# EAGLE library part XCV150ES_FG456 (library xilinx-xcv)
xcv150es_fg456 edit this description Auto generated by make-symbol-device-package-bsdl.ulp Rev. 26 Source: xcv150es_fg456.bsd
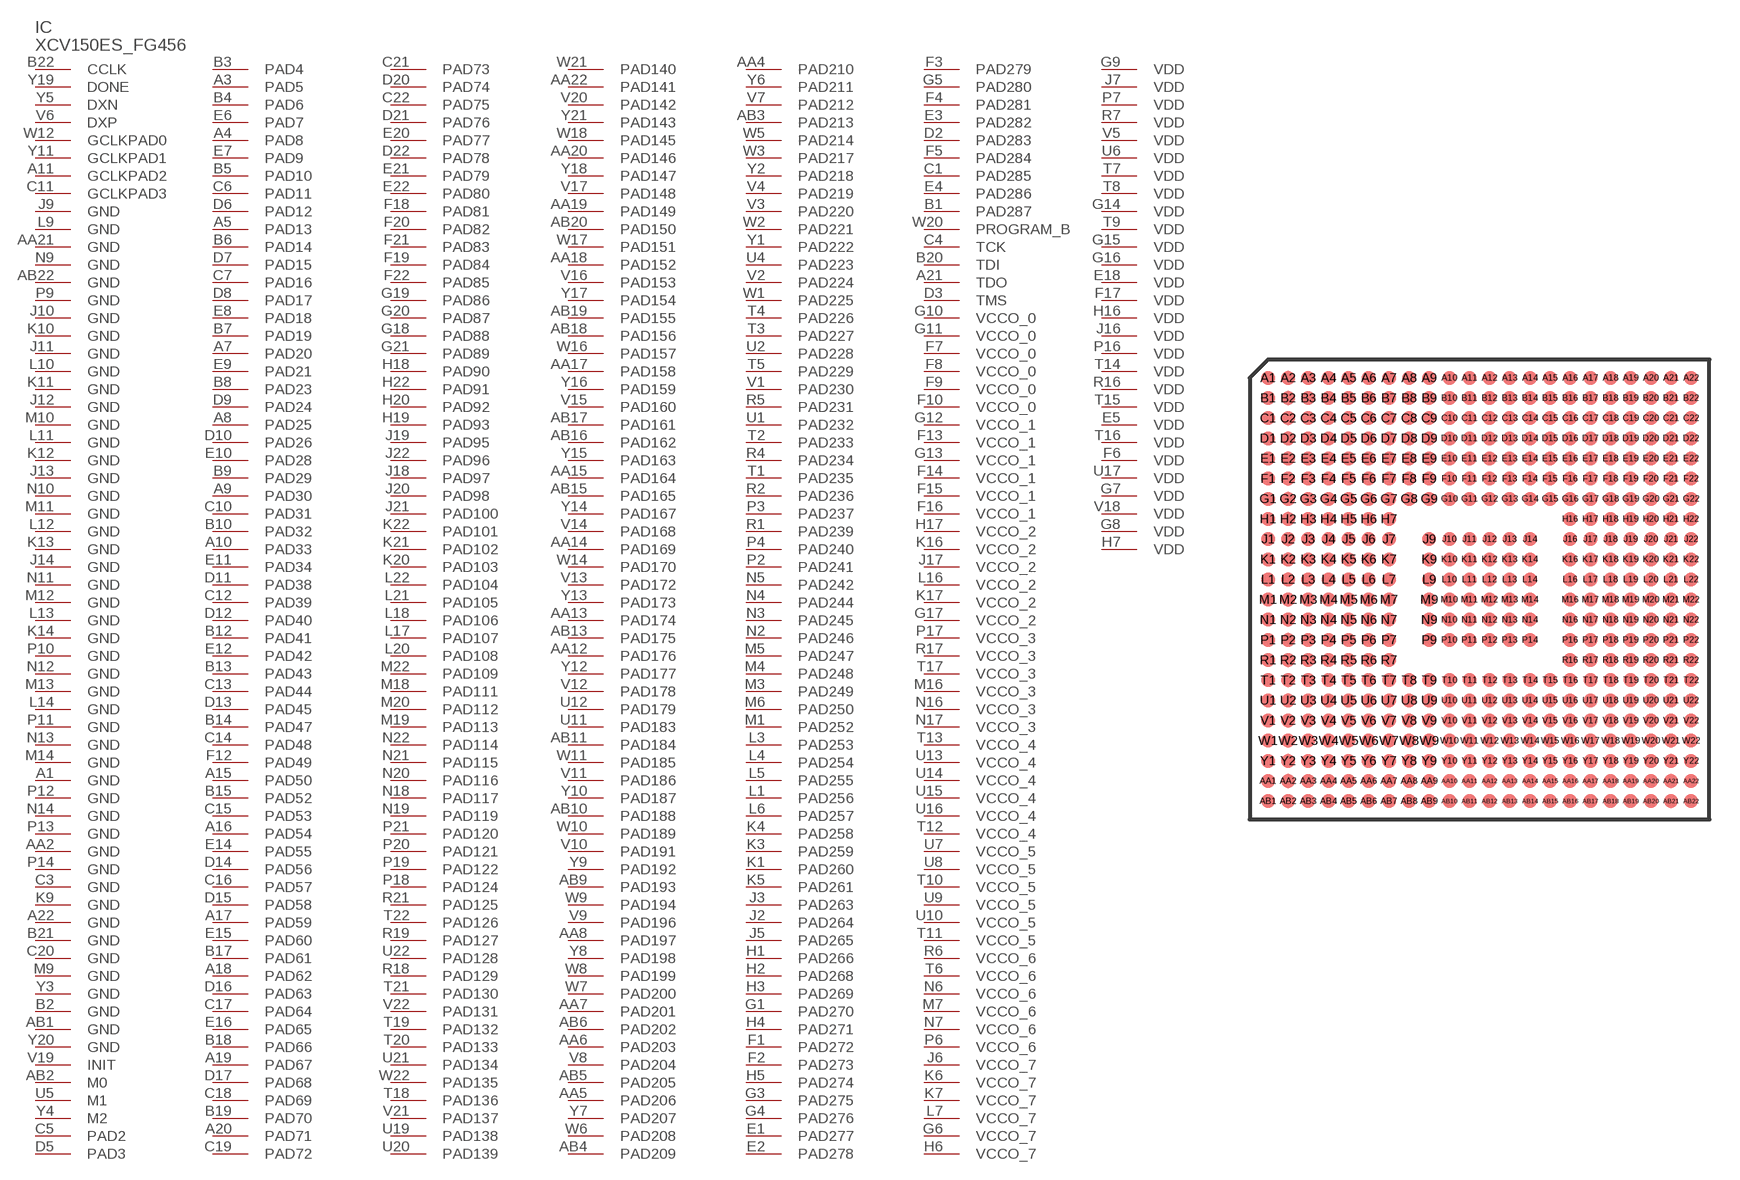
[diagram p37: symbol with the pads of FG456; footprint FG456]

Designator prefix IC

## XCV150ES_FG456 (OC_FARNELL: unknown; OC_NEWARK: unknown)  [FG456]
A1  GND  pwr
A3  PAD5
A4  PAD8
A5  PAD13
A7  PAD20
A8  PAD25
A9  PAD30
A10  PAD33
A11  GCLKPAD2  in
A15  PAD50
A16  PAD54
A17  PAD59
A18  PAD62
A19  PAD67
A20  PAD71
A21  TDO  out
A22  GND  pwr
AA2  GND  pwr
AA4  PAD210
AA5  PAD206
AA6  PAD203
AA7  PAD201
AA8  PAD197
AA12  PAD176
AA13  PAD174
AA14  PAD169
AA15  PAD164
AA17  PAD158
AA18  PAD152
AA19  PAD149
AA20  PAD146
AA21  GND  pwr
AA22  PAD141
AB1  GND  pwr
AB2  M0  in
AB3  PAD213
AB4  PAD209
AB5  PAD205
AB6  PAD202
AB9  PAD193
AB10  PAD188
AB11  PAD184
AB13  PAD175
AB15  PAD165
AB16  PAD162
AB17  PAD161
AB18  PAD156
AB19  PAD155
AB20  PAD150
AB22  GND  pwr
B1  PAD287
B2  GND  pwr
B3  PAD4
B4  PAD6
B5  PAD10
B6  PAD14
B7  PAD19
B8  PAD23
B9  PAD29
B10  PAD32
B12  PAD41
B13  PAD43
B14  PAD47
B15  PAD52
B17  PAD61
B18  PAD66
B19  PAD70
B20  TDI  in
B21  GND  pwr
B22  CCLK
C1  PAD285
C3  GND  pwr
C4  TCK  in
C5  PAD2
C6  PAD11
C7  PAD16
C10  PAD31
C11  GCLKPAD3  in
C12  PAD39
C13  PAD44
C14  PAD48
C15  PAD53
C16  PAD57
C17  PAD64
C18  PAD69
C19  PAD72
C20  GND  pwr
C21  PAD73
C22  PAD75
D2  PAD283
D3  TMS  in
D5  PAD3
D6  PAD12
D7  PAD15
D8  PAD17
D9  PAD24
D10  PAD26
D11  PAD38
D12  PAD40
D13  PAD45
D14  PAD56
D15  PAD58
D16  PAD63
D17  PAD68
D20  PAD74
D21  PAD76
D22  PAD78
E1  PAD277
E2  PAD278
E3  PAD282
E4  PAD286
E5  VDD  pwr
E6  PAD7
E7  PAD9
E8  PAD18
E9  PAD21
E10  PAD28
E11  PAD34
E12  PAD42
E14  PAD55
E15  PAD60
E16  PAD65
E18  VDD  pwr
E20  PAD77
E21  PAD79
E22  PAD80
F1  PAD272
F2  PAD273
F3  PAD279
F4  PAD281
F5  PAD284
F6  VDD  pwr
F7  VCCO_0  pwr
F8  VCCO_0  pwr
F9  VCCO_0  pwr
F10  VCCO_0  pwr
F12  PAD49
F13  VCCO_1  pwr
F14  VCCO_1  pwr
F15  VCCO_1  pwr
F16  VCCO_1  pwr
F17  VDD  pwr
F18  PAD81
F19  PAD84
F20  PAD82
F21  PAD83
F22  PAD85
G1  PAD270
G3  PAD275
G4  PAD276
G5  PAD280
G6  VCCO_7  pwr
G7  VDD  pwr
G8  VDD  pwr
G9  VDD  pwr
G10  VCCO_0  pwr
G11  VCCO_0  pwr
G12  VCCO_1  pwr
G13  VCCO_1  pwr
G14  VDD  pwr
G15  VDD  pwr
G16  VDD  pwr
G17  VCCO_2  pwr
G18  PAD88
G19  PAD86
G20  PAD87
G21  PAD89
H1  PAD266
H2  PAD268
H3  PAD269
H4  PAD271
H5  PAD274
H6  VCCO_7  pwr
H7  VDD  pwr
H16  VDD  pwr
H17  VCCO_2  pwr
H18  PAD90
H19  PAD93
H20  PAD92
H22  PAD91
J2  PAD264
J3  PAD263
J5  PAD265
J6  VCCO_7  pwr
J7  VDD  pwr
J9  GND  pwr
J10  GND  pwr
J11  GND  pwr
J12  GND  pwr
J13  GND  pwr
J14  GND  pwr
J16  VDD  pwr
J17  VCCO_2  pwr
J18  PAD97
J19  PAD95
J20  PAD98
J21  PAD100
J22  PAD96
K1  PAD260
K3  PAD259
K4  PAD258
K5  PAD261
K6  VCCO_7  pwr
K7  VCCO_7  pwr
K9  GND  pwr
K10  GND  pwr
K11  GND  pwr
K12  GND  pwr
K13  GND  pwr
K14  GND  pwr
K16  VCCO_2  pwr
K17  VCCO_2  pwr
K20  PAD103
K21  PAD102
K22  PAD101
L1  PAD256
L3  PAD253
L4  PAD254
L5  PAD255
L6  PAD257
L7  VCCO_7  pwr
L9  GND  pwr
L10  GND  pwr
L11  GND  pwr
L12  GND  pwr
L13  GND  pwr
L14  GND  pwr
L16  VCCO_2  pwr
L17  PAD107
L18  PAD106
L20  PAD108
L21  PAD105
L22  PAD104
M1  PAD252
M3  PAD249
M4  PAD248
M5  PAD247
M6  PAD250
M7  VCCO_6  pwr
M9  GND  pwr
M10  GND  pwr
M11  GND  pwr
M12  GND  pwr
M13  GND  pwr
M14  GND  pwr
M16  VCCO_3  pwr
M18  PAD111
M19  PAD113
M20  PAD112
M22  PAD109
N2  PAD246
N3  PAD245
N4  PAD244
N5  PAD242
N6  VCCO_6  pwr
N7  VCCO_6  pwr
N9  GND  pwr
N10  GND  pwr
N11  GND  pwr
N12  GND  pwr
N13  GND  pwr
N14  GND  pwr
N16  VCCO_3  pwr
N17  VCCO_3  pwr
N18  PAD117
N19  PAD119
N20  PAD116
N21  PAD115
N22  PAD114
P2  PAD241
P3  PAD237
P4  PAD240
P6  VCCO_6  pwr
P7  VDD  pwr
P9  GND  pwr
P10  GND  pwr
P11  GND  pwr
P12  GND  pwr
P13  GND  pwr
P14  GND  pwr
P16  VDD  pwr
P17  VCCO_3  pwr
P18  PAD124
P19  PAD122
P20  PAD121
P21  PAD120
R1  PAD239
R2  PAD236
R4  PAD234
R5  PAD231
R6  VCCO_6  pwr
R7  VDD  pwr
R16  VDD  pwr
R17  VCCO_3  pwr
R18  PAD129
R19  PAD127
R21  PAD125
T1  PAD235
T2  PAD233
T3  PAD227
T4  PAD226
T5  PAD229
T6  VCCO_6  pwr
T7  VDD  pwr
T8  VDD  pwr
T9  VDD  pwr
T10  VCCO_5  pwr
T11  VCCO_5  pwr
T12  VCCO_4  pwr
T13  VCCO_4  pwr
T14  VDD  pwr
T15  VDD  pwr
T16  VDD  pwr
T17  VCCO_3  pwr
T18  PAD136
T19  PAD132
T20  PAD133
T21  PAD130
T22  PAD126
U1  PAD232
U2  PAD228
U4  PAD223
U5  M1  in
U6  VDD  pwr
U7  VCCO_5  pwr
U8  VCCO_5  pwr
U9  VCCO_5  pwr
U10  VCCO_5  pwr
U11  PAD183
U12  PAD179
U13  VCCO_4  pwr
U14  VCCO_4  pwr
U15  VCCO_4  pwr
U16  VCCO_4  pwr
U17  VDD  pwr
U19  PAD138
U20  PAD139
U21  PAD134
U22  PAD128
V1  PAD230
V2  PAD224
V3  PAD220
V4  PAD219
V5  VDD  pwr
V6  DXP  pas
V7  PAD212
V8  PAD204
V9  PAD196
V10  PAD191
V11  PAD186
V12  PAD178
V13  PAD172
V14  PAD168
V15  PAD160
V16  PAD153
V17  PAD148
V18  VDD  pwr
V19  INIT
V20  PAD142
V21  PAD137
V22  PAD131
W1  PAD225
W2  PAD221
W3  PAD217
W5  PAD214
W6  PAD208
W7  PAD200
W8  PAD199
W9  PAD194
W10  PAD189
W11  PAD185
W12  GCLKPAD0  in
W14  PAD170
W16  PAD157
W17  PAD151
W18  PAD145
W20  PROGRAM_B  in
W21  PAD140
W22  PAD135
Y1  PAD222
Y2  PAD218
Y3  GND  pwr
Y4  M2  in
Y5  DXN  pas
Y6  PAD211
Y7  PAD207
Y8  PAD198
Y9  PAD192
Y10  PAD187
Y11  GCLKPAD1  in
Y12  PAD177
Y13  PAD173
Y14  PAD167
Y15  PAD163
Y16  PAD159
Y17  PAD154
Y18  PAD147
Y19  DONE
Y20  GND  pwr
Y21  PAD143

## Footprint FG456 (pad centres in mm)
xcv150_fg456 edit this description Auto generated by make-symbol-device-package-bsdl.ulp Rev. 26 Source: xcv150_fg456.bsd
smd 0.7 x 0.7: A1 -10.5,10.5; A2 -9.5,10.5; A3 -8.5,10.5; A4 -7.5,10.5; A5 -6.5,10.5; A6 -5.5,10.5; A7 -4.5,10.5; A8 -3.5,10.5; A9 -2.5,10.5; A10 -1.5,10.5; A11 -0.5,10.5; A12 0.5,10.5; A13 1.5,10.5; A14 2.5,10.5; A15 3.5,10.5; A16 4.5,10.5; A17 5.5,10.5; A18 6.5,10.5; A19 7.5,10.5; A20 8.5,10.5; A21 9.5,10.5; A22 10.5,10.5; AA1 -10.5,-9.5; AA2 -9.5,-9.5; AA3 -8.5,-9.5; AA4 -7.5,-9.5; AA5 -6.5,-9.5; AA6 -5.5,-9.5; AA7 -4.5,-9.5; AA8 -3.5,-9.5; AA9 -2.5,-9.5; AA10 -1.5,-9.5; AA11 -0.5,-9.5; AA12 0.5,-9.5; AA13 1.5,-9.5; AA14 2.5,-9.5; AA15 3.5,-9.5; AA16 4.5,-9.5; AA17 5.5,-9.5; AA18 6.5,-9.5; AA19 7.5,-9.5; AA20 8.5,-9.5; AA21 9.5,-9.5; AA22 10.5,-9.5; AB1 -10.5,-10.5; AB2 -9.5,-10.5; AB3 -8.5,-10.5; AB4 -7.5,-10.5; AB5 -6.5,-10.5; AB6 -5.5,-10.5; AB7 -4.5,-10.5; AB8 -3.5,-10.5; AB9 -2.5,-10.5; AB10 -1.5,-10.5; AB11 -0.5,-10.5; AB12 0.5,-10.5; AB13 1.5,-10.5; AB14 2.5,-10.5; AB15 3.5,-10.5; AB16 4.5,-10.5; AB17 5.5,-10.5; AB18 6.5,-10.5; AB19 7.5,-10.5; AB20 8.5,-10.5; AB21 9.5,-10.5; AB22 10.5,-10.5; B1 -10.5,9.5; B2 -9.5,9.5; B3 -8.5,9.5; B4 -7.5,9.5; B5 -6.5,9.5; B6 -5.5,9.5; B7 -4.5,9.5; B8 -3.5,9.5; B9 -2.5,9.5; B10 -1.5,9.5; B11 -0.5,9.5; B12 0.5,9.5; B13 1.5,9.5; B14 2.5,9.5; B15 3.5,9.5; B16 4.5,9.5; B17 5.5,9.5; B18 6.5,9.5; B19 7.5,9.5; B20 8.5,9.5; B21 9.5,9.5; B22 10.5,9.5; C1 -10.5,8.5; C2 -9.5,8.5; C3 -8.5,8.5; C4 -7.5,8.5; C5 -6.5,8.5; C6 -5.5,8.5; C7 -4.5,8.5; C8 -3.5,8.5; C9 -2.5,8.5; C10 -1.5,8.5; C11 -0.5,8.5; C12 0.5,8.5; C13 1.5,8.5; C14 2.5,8.5; C15 3.5,8.5; C16 4.5,8.5; C17 5.5,8.5; C18 6.5,8.5; C19 7.5,8.5; C20 8.5,8.5; C21 9.5,8.5; C22 10.5,8.5; D1 -10.5,7.5; D2 -9.5,7.5; D3 -8.5,7.5; D4 -7.5,7.5; D5 -6.5,7.5; D6 -5.5,7.5; D7 -4.5,7.5; D8 -3.5,7.5; D9 -2.5,7.5; D10 -1.5,7.5; D11 -0.5,7.5; D12 0.5,7.5; D13 1.5,7.5; D14 2.5,7.5; D15 3.5,7.5; D16 4.5,7.5; D17 5.5,7.5; D18 6.5,7.5; D19 7.5,7.5; D20 8.5,7.5; D21 9.5,7.5; D22 10.5,7.5; E1 -10.5,6.5; E2 -9.5,6.5; E3 -8.5,6.5; E4 -7.5,6.5; E5 -6.5,6.5; E6 -5.5,6.5; E7 -4.5,6.5; E8 -3.5,6.5; E9 -2.5,6.5; E10 -1.5,6.5; E11 -0.5,6.5; E12 0.5,6.5; E13 1.5,6.5; E14 2.5,6.5; E15 3.5,6.5; E16 4.5,6.5; E17 5.5,6.5; E18 6.5,6.5; E19 7.5,6.5; E20 8.5,6.5; E21 9.5,6.5; E22 10.5,6.5; F1 -10.5,5.5; F2 -9.5,5.5; F3 -8.5,5.5; F4 -7.5,5.5; F5 -6.5,5.5; F6 -5.5,5.5; F7 -4.5,5.5; F8 -3.5,5.5; F9 -2.5,5.5; F10 -1.5,5.5; F11 -0.5,5.5; F12 0.5,5.5; F13 1.5,5.5; F14 2.5,5.5; F15 3.5,5.5; F16 4.5,5.5; F17 5.5,5.5; F18 6.5,5.5; F19 7.5,5.5; F20 8.5,5.5; F21 9.5,5.5; F22 10.5,5.5; G1 -10.5,4.5; G2 -9.5,4.5; G3 -8.5,4.5; G4 -7.5,4.5; G5 -6.5,4.5; G6 -5.5,4.5; G7 -4.5,4.5; G8 -3.5,4.5; G9 -2.5,4.5; G10 -1.5,4.5; G11 -0.5,4.5; G12 0.5,4.5; G13 1.5,4.5; G14 2.5,4.5; G15 3.5,4.5; G16 4.5,4.5; G17 5.5,4.5; G18 6.5,4.5; G19 7.5,4.5; G20 8.5,4.5; G21 9.5,4.5; G22 10.5,4.5; H1 -10.5,3.5; H2 -9.5,3.5; H3 -8.5,3.5; H4 -7.5,3.5; H5 -6.5,3.5; H6 -5.5,3.5; H7 -4.5,3.5; H16 4.5,3.5; H17 5.5,3.5; H18 6.5,3.5; H19 7.5,3.5; H20 8.5,3.5; H21 9.5,3.5; H22 10.5,3.5; J1 -10.5,2.5; J2 -9.5,2.5; J3 -8.5,2.5; J4 -7.5,2.5; J5 -6.5,2.5; J6 -5.5,2.5; J7 -4.5,2.5; J9 -2.5,2.5; J10 -1.5,2.5; J11 -0.5,2.5; J12 0.5,2.5; J13 1.5,2.5; J14 2.5,2.5; J16 4.5,2.5; J17 5.5,2.5; J18 6.5,2.5; J19 7.5,2.5; J20 8.5,2.5; J21 9.5,2.5; J22 10.5,2.5; K1 -10.5,1.5; K2 -9.5,1.5; K3 -8.5,1.5; K4 -7.5,1.5; K5 -6.5,1.5; K6 -5.5,1.5; K7 -4.5,1.5; K9 -2.5,1.5; K10 -1.5,1.5; K11 -0.5,1.5; K12 0.5,1.5; K13 1.5,1.5; K14 2.5,1.5; K16 4.5,1.5; K17 5.5,1.5; K18 6.5,1.5; K19 7.5,1.5; K20 8.5,1.5; K21 9.5,1.5; K22 10.5,1.5; L1 -10.5,0.5; L2 -9.5,0.5; L3 -8.5,0.5; L4 -7.5,0.5; L5 -6.5,0.5; L6 -5.5,0.5; L7 -4.5,0.5; L9 -2.5,0.5; L10 -1.5,0.5; L11 -0.5,0.5; L12 0.5,0.5; L13 1.5,0.5; L14 2.5,0.5; L16 4.5,0.5; L17 5.5,0.5; L18 6.5,0.5; L19 7.5,0.5; L20 8.5,0.5; L21 9.5,0.5; L22 10.5,0.5; M1 -10.5,-0.5; M2 -9.5,-0.5; M3 -8.5,-0.5; M4 -7.5,-0.5; M5 -6.5,-0.5; M6 -5.5,-0.5; M7 -4.5,-0.5; M9 -2.5,-0.5; M10 -1.5,-0.5; M11 -0.5,-0.5; M12 0.5,-0.5; M13 1.5,-0.5; M14 2.5,-0.5; M16 4.5,-0.5; M17 5.5,-0.5; M18 6.5,-0.5; M19 7.5,-0.5; M20 8.5,-0.5; M21 9.5,-0.5; M22 10.5,-0.5; N1 -10.5,-1.5; N2 -9.5,-1.5; N3 -8.5,-1.5; N4 -7.5,-1.5; N5 -6.5,-1.5; N6 -5.5,-1.5; N7 -4.5,-1.5; N9 -2.5,-1.5; N10 -1.5,-1.5; N11 -0.5,-1.5; N12 0.5,-1.5; N13 1.5,-1.5; N14 2.5,-1.5; N16 4.5,-1.5; N17 5.5,-1.5; N18 6.5,-1.5; N19 7.5,-1.5; N20 8.5,-1.5; N21 9.5,-1.5; N22 10.5,-1.5; P1 -10.5,-2.5; P2 -9.5,-2.5; P3 -8.5,-2.5; P4 -7.5,-2.5; P5 -6.5,-2.5; P6 -5.5,-2.5; P7 -4.5,-2.5; P9 -2.5,-2.5; P10 -1.5,-2.5; P11 -0.5,-2.5; P12 0.5,-2.5; P13 1.5,-2.5; P14 2.5,-2.5; P16 4.5,-2.5; P17 5.5,-2.5; P18 6.5,-2.5; P19 7.5,-2.5; P20 8.5,-2.5; P21 9.5,-2.5; P22 10.5,-2.5; R1 -10.5,-3.5; R2 -9.5,-3.5; R3 -8.5,-3.5; R4 -7.5,-3.5; R5 -6.5,-3.5; R6 -5.5,-3.5; R7 -4.5,-3.5; R16 4.5,-3.5; R17 5.5,-3.5; R18 6.5,-3.5; R19 7.5,-3.5; R20 8.5,-3.5; R21 9.5,-3.5; R22 10.5,-3.5; T1 -10.5,-4.5; T2 -9.5,-4.5; T3 -8.5,-4.5; T4 -7.5,-4.5; T5 -6.5,-4.5; T6 -5.5,-4.5; T7 -4.5,-4.5; T8 -3.5,-4.5; T9 -2.5,-4.5; T10 -1.5,-4.5; T11 -0.5,-4.5; T12 0.5,-4.5; T13 1.5,-4.5; T14 2.5,-4.5; T15 3.5,-4.5; T16 4.5,-4.5; T17 5.5,-4.5; T18 6.5,-4.5; T19 7.5,-4.5; T20 8.5,-4.5; T21 9.5,-4.5; T22 10.5,-4.5; U1 -10.5,-5.5; U2 -9.5,-5.5; U3 -8.5,-5.5; U4 -7.5,-5.5; U5 -6.5,-5.5; U6 -5.5,-5.5; U7 -4.5,-5.5; U8 -3.5,-5.5; U9 -2.5,-5.5; U10 -1.5,-5.5; U11 -0.5,-5.5; U12 0.5,-5.5; U13 1.5,-5.5; U14 2.5,-5.5; U15 3.5,-5.5; U16 4.5,-5.5; U17 5.5,-5.5; U18 6.5,-5.5; U19 7.5,-5.5; U20 8.5,-5.5; U21 9.5,-5.5; U22 10.5,-5.5; V1 -10.5,-6.5; V2 -9.5,-6.5; V3 -8.5,-6.5; V4 -7.5,-6.5; V5 -6.5,-6.5; V6 -5.5,-6.5; V7 -4.5,-6.5; V8 -3.5,-6.5; V9 -2.5,-6.5; V10 -1.5,-6.5; V11 -0.5,-6.5; V12 0.5,-6.5; V13 1.5,-6.5; V14 2.5,-6.5; V15 3.5,-6.5; V16 4.5,-6.5; V17 5.5,-6.5; V18 6.5,-6.5; V19 7.5,-6.5; V20 8.5,-6.5; V21 9.5,-6.5; V22 10.5,-6.5; W1 -10.5,-7.5; W2 -9.5,-7.5; W3 -8.5,-7.5; W4 -7.5,-7.5; W5 -6.5,-7.5; W6 -5.5,-7.5; W7 -4.5,-7.5; W8 -3.5,-7.5; W9 -2.5,-7.5; W10 -1.5,-7.5; W11 -0.5,-7.5; W12 0.5,-7.5; W13 1.5,-7.5; W14 2.5,-7.5; W15 3.5,-7.5; W16 4.5,-7.5; W17 5.5,-7.5; W18 6.5,-7.5; W19 7.5,-7.5; W20 8.5,-7.5; W21 9.5,-7.5; W22 10.5,-7.5; Y1 -10.5,-8.5; Y2 -9.5,-8.5; Y3 -8.5,-8.5; Y4 -7.5,-8.5; Y5 -6.5,-8.5; Y6 -5.5,-8.5; Y7 -4.5,-8.5; Y8 -3.5,-8.5; Y9 -2.5,-8.5; Y10 -1.5,-8.5; Y11 -0.5,-8.5; Y12 0.5,-8.5; Y13 1.5,-8.5; Y14 2.5,-8.5; Y15 3.5,-8.5; Y16 4.5,-8.5; Y17 5.5,-8.5; Y18 6.5,-8.5; Y19 7.5,-8.5; Y20 8.5,-8.5; Y21 9.5,-8.5; Y22 10.5,-8.5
